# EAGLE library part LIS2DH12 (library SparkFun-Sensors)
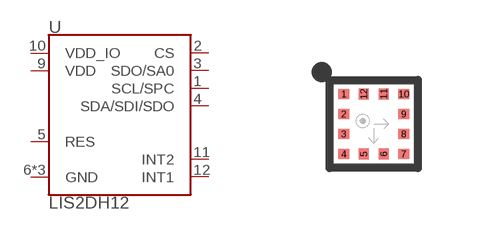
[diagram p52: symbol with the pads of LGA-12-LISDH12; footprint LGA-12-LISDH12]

Designator prefix U

## LIS2DH12 (DIGIKEY: 497-14851-2-ND; PROD_ID: IC-14229)  [LGA-12-LISDH12]
1  SCL/SPC
2  CS
3  SDO/SA0
4  SDA/SDI/SDO
5  RES
6  GND
7  GND
8  GND
9  VDD
10  VDD_IO
11  INT2
12  INT1

## Footprint LGA-12-LISDH12 (pad centres in mm)
smd 0.275 x 0.25: 1 -0.75,0.75; 2 -0.75,0.25; 3 -0.75,-0.25; 4 -0.75,-0.75; 7 0.75,-0.75; 8 0.75,-0.25; 9 0.75,0.25; 10 0.75,0.75
smd 0.25 x 0.275: 5 -0.25,-0.75; 6 0.25,-0.75; 11 0.25,0.75; 12 -0.25,0.75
